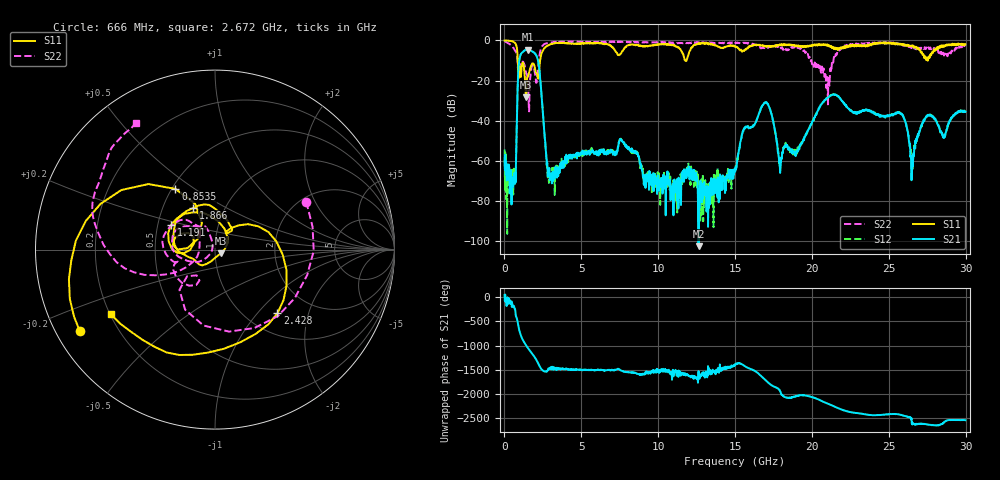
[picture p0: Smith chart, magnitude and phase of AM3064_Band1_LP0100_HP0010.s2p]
# Hz S DB R 50.0
!freq dBS11 angS11 dBS21 angS21 dBS12 angS12 dBS22 angS22
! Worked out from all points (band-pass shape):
!   1600 points, 10 MHz to 29.98 GHz, reference 50 ohm
!   highest |S21| = -4.52 dB at 1.51 GHz (marker M1); lowest = -102.5 dB at 12.62 GHz (marker M2)
!   |S21| within 3 dB of the highest: 1.033 GHz to 2.077 GHz (1.044 GHz wide, 67.1 % of centre)
!   lowest |S11| = -28.4 dB at 1.397 GHz (marker M3), VSWR 1.08, Z = 53.2 - j2.28 ohm
!   |S11| at or under -10 dB: 865.7 MHz to 2.317 GHz (1.451 GHz wide, 91.2 % of centre); 11.76 GHz to 11.84 GHz (88.3 MHz wide, 0.748 % of centre); 27.52339 GHz to 27.53514 GHz (11.75 MHz wide, 0.0427 % of centre)
!   |S22| runs from -35.3 to -0.4 dB; largest |S21 - S12| = 0.009
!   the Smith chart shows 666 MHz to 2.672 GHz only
!   S11 on the Smith chart (normalised r, x): 666 MHz: 0.07, -0.28; 853.5 MHz: 0.52, +0.42; 1.191 GHz: 0.59, +0.17; 1.866 GHz: 0.71, +0.35; 2.428 GHz: 1.36, -1.29; 2.672 GHz: 0.20, -0.27
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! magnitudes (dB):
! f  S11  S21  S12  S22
! 10 MHz  0.0  -58.4  -54.3  -0.4
! 666 MHz  -1.1  -66.6  -67.4  -4.8
! 853.5 MHz  -7.9  -24.8  -24.7  -10.5
! 1.191 GHz  -11.0  -5.8  -5.7  -10.6
! 1.397 GHz  -28.4  -4.6  -4.6  -16.0
! 1.51 GHz  -18.2  -4.5  -4.5  -19.5
! 1.866 GHz  -11.6  -5.8  -5.8  -12.2
! 2.428 GHz  -6.1  -28.9  -28.9  -3.1
! 2.672 GHz  -3.3  -53.0  -53.3  -1.6
! 3.103 GHz  -1.8  -65.9  -63.5  -1.0
! 5.015 GHz  -1.5  -56.5  -56.8  -0.7
! 7.639 GHz  -5.6  -50.0  -49.5  -0.7
! 10 GHz  -2.0  -67.2  -68.4  -1.0
! 12.62 GHz  -1.5  -102.5  -69.9  -0.9
! 15 GHz  -3.1  -65.3  -64.2  -1.5
! 16.92 GHz  -2.8  -31.1  -31.1  -3.9
! 17.93 GHz  -2.0  -66.0  -63.9  -3.1
! 19.99 GHz  -2.8  -41.3  -41.2  -11.2
! 25 GHz  -1.1  -37.6  -37.3  -1.2
! 26.55 GHz  -2.4  -61.5  -64.0  -4.3
! 27.51 GHz  -9.4  -37.6  -37.2  -4.4
! 29.98 GHz  -1.9  -35.5  -35.1  -2.9
